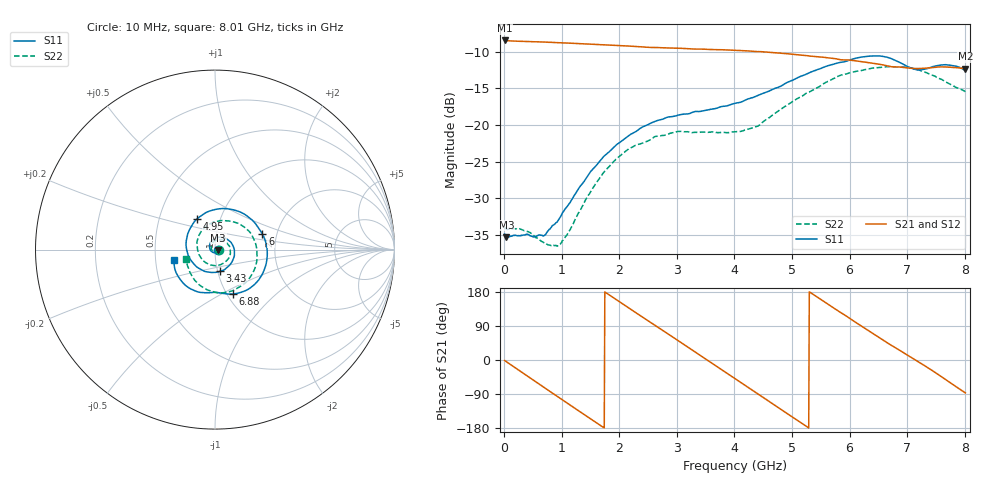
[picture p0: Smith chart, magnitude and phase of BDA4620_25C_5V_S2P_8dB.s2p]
!Agilent Technologies,E5071B,MY42404982,A.09.10
!Date: Wed May 06 08:59:48 2026
!Data & Calibration Information:
!Freq	S11:SOLT2(ON)	S21:SOLT2(ON)	S12:SOLT2(ON)	S22:SOLT2(ON)
# Hz S RI R 50
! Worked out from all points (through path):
!   801 points, 10 MHz to 8.01 GHz, reference 50 ohm
!   highest |S21| = -8.44 dB at 10 MHz (marker M1); lowest = -12.3 dB at 8.01 GHz (marker M2)
!   group delay of S21, straight-line fit = 280 ps
!   lowest |S11| = -35.3 dB at 40 MHz (marker M3), VSWR 1.03, Z = 51.7 - j0.199 ohm
!   |S11| at or under -10 dB: start of sweep to end of sweep
!   |S22| runs from -36.6 to -12.0 dB; largest |S21 - S12| = 0.0016
!   S11 on the Smith chart (normalised r, x): 10 MHz: 1.04, -0.00; 3.43 GHz: 1.02, -0.25; 4.95 GHz: 0.77, +0.27; 6 GHz: 1.68, +0.31; 6.88 GHz: 1.06, -0.57; 8.01 GHz: 0.62, -0.08
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1e7  0.0179 -0.00134  0.3784 -0.00817  0.3787 -0.00827  0.0199 -0.00122
4e7  0.017 -0.00193  0.3761 -0.0282  0.3767 -0.0296  0.0194 -0.00159
3.6e8  0.012 -0.0131  0.295 -0.2279  0.295 -0.2286  0.0154 -0.0109
7.3e8  -0.00702 -0.0167  0.0893 -0.3574  0.0892 -0.3579  -8.82e-05 -0.0155
9.6e8  -0.0214 -0.0083  -0.0613 -0.3601  -0.0616 -0.3605  -0.012 -0.00924
1.35e9  -0.0301 0.0253  -0.2742 -0.2327  -0.2744 -0.2329  -0.0211 0.0174
1.65e9  -0.0123 0.0544  -0.3493 -0.0598  -0.3499 -0.0601  -0.00963 0.0416
1.94e9  0.0227 0.069  -0.3292 0.1182  -0.3299 0.1185  0.0173 0.0555
2.32e9  0.0761 0.0515  -0.1801 0.2927  -0.1806 0.2931  0.0591 0.0439
2.68e9  0.1078 -0.00189  0.0259 0.3373  0.0264 0.3377  0.0836 0.00775
3.01e9  0.0959 -0.0656  0.2045 0.2654  0.2051 0.2657  0.0822 -0.0375
3.43e9  0.0274 -0.1213  0.3252 0.0578  0.3257 0.0575  0.0355 -0.0822
4.01e9  -0.1053 -0.0931  0.2131 -0.2442  0.2132 -0.2447  -0.0635 -0.0637
4.47e9  -0.1611 0.0255  -0.0318 -0.3156  -0.032 -0.316  -0.1 0.0235
4.95e9  -0.1016 0.1699  -0.25 -0.1767  -0.2504 -0.1768  -0.0459 0.1318
5.35e9  0.0393 0.2285  -0.2938 0.0264  -0.2942 0.0265  0.0628 0.1603
6e9  0.2641 0.0862  -0.0951 0.261  -0.0956 0.2613  0.2234 0.0419
6.33e9  0.2864 -0.0729  0.0601 0.2602  0.0608 0.2601  0.2318 -0.0685
6.68e9  0.1859 -0.2205  0.1852 0.1711  0.1857 0.1715  0.175 -0.1793
6.88e9  0.0989 -0.2474  0.2268 0.1019  0.2276 0.1022  0.1172 -0.2198
7.44e9  -0.0719 -0.2398  0.2174 -0.1172  0.218 -0.1175  -0.0759 -0.2052
8.01e9  -0.2283 -0.0588  0.0129 -0.242  0.0129 -0.2425  -0.1604 -0.0528
